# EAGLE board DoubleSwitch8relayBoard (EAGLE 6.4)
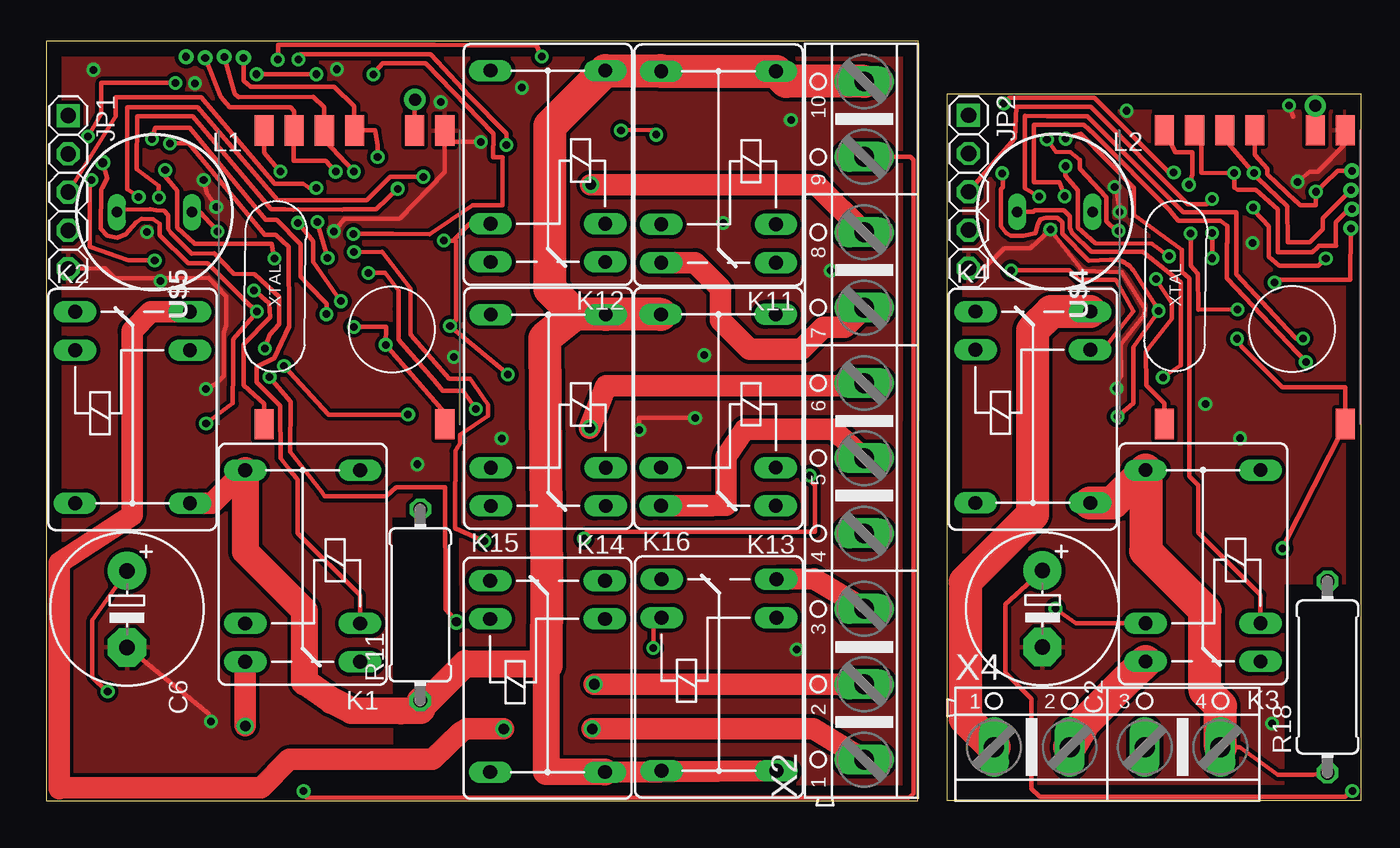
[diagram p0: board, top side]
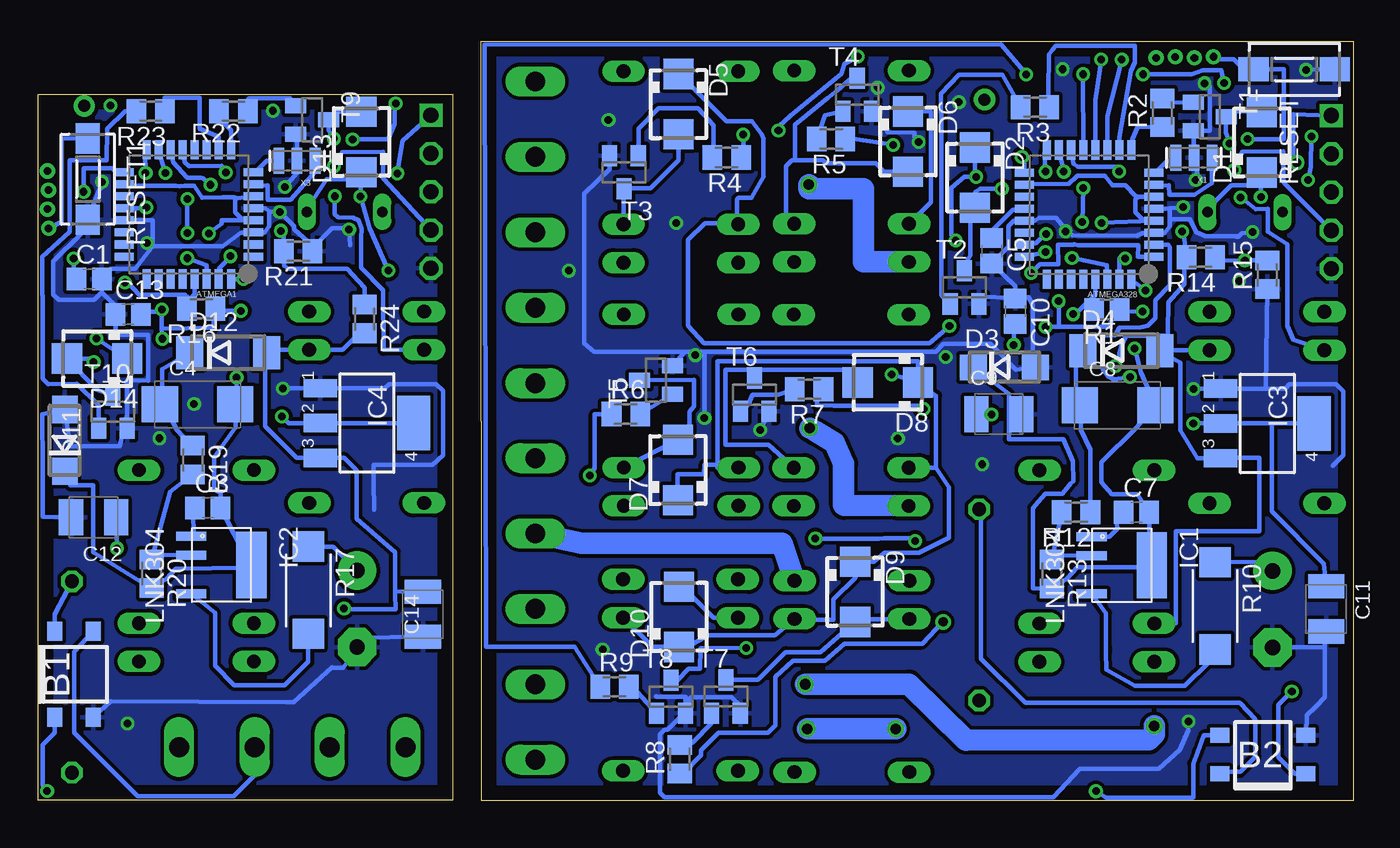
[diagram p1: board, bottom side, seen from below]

Size 87.28 x 50.4 mm. Coordinates in mm from the lower left corner, seen from the top.
Outline: 59.78,46.89 87.28,46.89 87.28,46.8 87.28,0.02 59.78,0.02 59.78,46.89
Outline: 0,0 57.85,0 57.9,50.38 0,50.4 0,0
Copper layers (1*16): Top 0.035mm / dielectric 1.5mm / Bottom 0.035mm
Design rules "default": minimum track width 10mil, minimum drill 24mil, track to track 8mil, track to pad 8mil, pad to pad 8mil, via to via 8mil, smd to smd 8mil, copper to edge 40mil, drill to drill 8mil, minimum pad ring 10mil, minimum via ring 8mil, stop-mask expansion 4mil, vias tented up to drill 0mil, thermal gap 10mil
Net classes: 1 power: width 0.381 mm, clearance 0.254 mm; 2 220V: width 0.381 mm, clearance 0.508 mm

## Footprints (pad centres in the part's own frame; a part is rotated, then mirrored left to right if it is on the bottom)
TQFP32-08 = smd 1.27 x 0.533: 1 -4.293,2.8; 2 -4.293,2; 3 -4.293,1.2; 4 -4.293,0.4; 5 -4.293,-0.4; 6 -4.293,-1.2; 7 -4.293,-2; 8 -4.293,-2.8; 17 4.293,-2.8; 18 4.293,-2; 19 4.293,-1.2; 20 4.293,-0.4; 21 4.293,0.4; 22 4.293,1.2; 23 4.293,2; 24 4.293,2.8 | smd 0.533 x 1.27: 9 -2.8,-4.293; 10 -2,-4.293; 11 -1.2,-4.293; 12 -0.4,-4.293; 13 0.4,-4.293; 14 1.2,-4.293; 15 2,-4.293; 16 2.8,-4.293; 25 2.8,4.293; 26 2,4.293; 27 1.2,4.293; 28 0.4,4.293; 29 -0.4,4.293; 30 -1.2,4.293; 31 -2,4.293; 32 -2.8,4.293
TO-269AA = smd 1 x 1.25: + -1.28,-2.855; - 1.28,-2.855; AC1 -1.28,2.855; AC2 1.28,2.855
C2012 = smd 1.3 x 1.5: 1 -0.85,0; 2 0.85,0
E5-10,5 = drill 1.016 pad 2.54: + -2.54,0 | drill 1.016 pad 2.54 octagon: - 2.54,0
SMC_C = smd 2.4 x 2.4: + -2.5,0; - 2.5,0
SMC_B = smd 1.6 x 2.4: + -1.5,0; - 1.5,0
SMA = smd 2 x 2: A 2,0; C -2,0
DO214AC = smd 1.8 x 1.7: A 2.05,0; C -2.05,0
DO214AA = smd 1.8 x 2.2: A 2.55,0; C -2.55,0
SO-8C = smd 0.6 x 2: BP -1.905,-2; D 1.905,-2; FB -0.635,-2 | smd 4.41 x 2: S 0,2
SOT223 = smd 1.219 x 2.235: 1 -2.311,-3.099; 2 0,-3.099; 3 2.311,-3.099 | smd 3.6 x 2.2: 4 0,3.099
1X05-S = drill 1.016 square: 1 -5.08,0 | drill 1.016 octagon: 2 -2.54,0; 3 0,0; 4 2.54,0; 5 5.08,0
FRS1B = drill 0.914 long: 1 0,3.81; 2 0,-3.81; O -2.54,-3.81; P 10.16,3.81; P@ 10.16,-3.81; S -2.54,3.81
BS11 = drill 0.7 long: 1 -2.5,0; 2 2.5,0
R2012 = smd 1.3 x 1.5: 1 -0.85,0; 2 0.85,0
M2012 = smd 1.3 x 1.6: 1 -0.95,0; 2 0.95,0
R2512W = smd 2 x 2.1: 1 -2.896,0; 2 2.896,0
0411/12 = drill 0.914 octagon: 1 -6.35,0; 2 6.35,0
DTSM-3 = smd 2 x 1.6: 1 -2.7,0; 2 2.7,0
SOT23 = smd 1 x 1.4: 1 -0.95,-1.1; 2 0.95,-1.1; 3 0,1.1
RFM12B-ANTENNA = drill 0.8 pad 1.422: P$1 0,0
AVRHEADER = drill 0.5: CLK 2.54,0; MISO 1.27,0.07; MOSI 0,0; VPP -1.27,0.072
RFM69W-MINPADS = smd 2 x 1.27: ANA 8,-5; DIO0 -11.5,5; GND 8,-7; MISO 8,1; MOSI 8,3; NSS 8,5; SCK 8,-1; VDD -11.5,-7
RESONATOR-SMD = smd 0.7 x 1.7: 1 -1.2,0; 2 0,0; 3 1.2,0
AK500/10 = drill 1.321 long: 1 -22.504,0; 2 -17.501,0; 3 -12.497,0; 4 -7.493,0; 5 -2.489,0; 6 2.489,0; 7 7.493,0; 8 12.497,0; 9 17.501,0; 10 22.504,0
AK500/4 = drill 1.321 long: 1 -7.518,0; 2 -2.489,0; 3 2.489,0; 4 7.518,0

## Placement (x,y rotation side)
ATMEGA1  ATMega-328  [TQFP32-08]  77.29,38.9 180 bottom
ATMEGA328  ATMega-328  [TQFP32-08]  17.52,38.88 180 bottom
B1  RECTIFIER  [TO-269AA]  84.92,8.38 0 bottom
B2  RECTIFIER  [TO-269AA]  5.99,3.05 90 bottom
C1  0.1  [C2012]  83.91,34.61 0 bottom
C2  3,3uF  [E5-10,5]  66.12,12.73 270 top
C3  100nF  [C2012]  76.03,19.42 0 bottom
C4  22uF / 16 V  [SMC_C]  76.71,26.29 0 bottom
C5  0.1  [C2012]  23.99,36.48 270 bottom
C6  3,3uF  [E5-10,5]  5.35,12.7 270 top
C7  100nF  [C2012]  14.38,19.13 0 bottom
C8  22uF / 16 V  [SMC_C]  15.64,26.24 0 bottom
C9  100uF  [SMC_B]  23.51,25.65 0 bottom
C10  100nF  [C2012]  22.43,32.48 270 bottom
C11  100uF  [SMC_B]  1.79,12.72 270 bottom
C12  100uF  [SMC_B]  83.61,18.8 180 bottom
C13  100nF  [C2012]  81.32,32.27 0 bottom
C14  100uF  [SMC_B]  61.75,12.37 270 bottom
D1  MBRA340T3  [SMA]  6.06,43.68 90 bottom
D2  MBRA340T3  [SMA]  25.1,41.34 270 bottom
D3  ES1D  [DO214AC]  23.15,28.75 0 bottom
D4  1N4007GP  [DO214AA]  15.38,29.86 0 bottom
D5  MBRA340T3  [SMA]  44.79,46.22 270 bottom
D6  MBRA340T3  [SMA]  29.55,43.73 270 bottom
D7  MBRA340T3  [SMA]  44.82,21.94 90 bottom
D8  MBRA340T3  [SMA]  30.89,27.75 180 bottom
D9  MBRA340T3  [SMA]  33.05,13.85 270 bottom
D10  MBRA340T3  [SMA]  44.74,12.19 90 bottom
D11  ES1D  [DO214AC]  85.52,23.9 90 bottom
D12  1N4007GP  [DO214AA]  74.67,29.72 0 bottom
D13  MBRA340T3  [SMA]  65.83,43.7 90 bottom
D14  MBRA340T3  [SMA]  83.37,29.34 180 bottom
IC1  LNK304  [SO-8C]  15.35,15.62 270 bottom
IC2  LNK304  [SO-8C]  75.13,15.64 270 bottom
IC3  MC33269ST-3.3T3  [SOT223]  5.69,25.03 270 bottom
IC4  MC33269ST-3.3T3  [SOT223]  65.47,25.05 270 bottom
JP1  [1X05-S]  1.44,40.38 270 top
JP2  [1X05-S]  61.22,40.4 270 top
K1  FRS1B  [FRS1B]  17.01,11.75 90 top
K2  FRS1B  [FRS1B]  5.71,29.89 270 top
K3  FRS1B  [FRS1B]  76.78,11.78 90 top
K4  FRS1B  [FRS1B]  65.49,29.92 270 top
K11  FRS1B  [FRS1B]  44.62,38.24 90 top
K12  FRS1B  [FRS1B]  33.29,38.28 90 top
K13  FRS1B  [FRS1B]  44.61,22.1 90 top
K14  FRS1B  [FRS1B]  33.32,22.09 90 top
K15  FRS1B  [FRS1B]  33.27,12.05 270 top
K16  FRS1B  [FRS1B]  44.65,12.14 270 top
L1  680uH  [BS11]  7.17,39.05 0 top
L2  680uH  [BS11]  66.94,39.07 0 top
R1  10k  [R2012]  16.34,32.59 180 bottom
R2  1 K  [M2012]  12.67,45.64 90 bottom
R3  1 K  [M2012]  21.12,46.02 180 bottom
R4  1 K  [M2012]  41.58,42.68 180 bottom
R5  1 K  [M2012]  34.65,43.91 180 bottom
R6  1 K  [M2012]  48.28,25.65 0 bottom
R7  1 K  [M2012]  36.11,27.3 180 bottom
R8  1 K  [M2012]  44.69,2.74 90 bottom
R9  1 K  [M2012]  49.03,7.55 0 bottom
R10  100  [R2512W]  9.16,12.92 270 bottom
R11  8,2  [0411/12]  24.82,12.98 90 top
R12  3.9 k  [M2012]  18.39,19.14 180 bottom
R13  2,05 k  [M2012]  19.98,15.03 270 bottom
R14  470  [M2012]  10.11,36.05 180 bottom
R15  470  [M2012]  5.69,34.89 90 bottom
R16  10k  [M2012]  76.47,32.65 180 bottom
R17  100  [R2512W]  69.35,13.96 270 bottom
R18  8,2  [0411/12]  85.05,8.2 90 top
R19  3.9 k  [M2012]  77.02,22.6 270 bottom
R20  2,05 k  [M2012]  79.76,15.06 270 bottom
R21  560  [M2012]  70.03,36.46 180 bottom
R22  1 K  [M2012]  74.33,45.75 0 bottom
R23  1 K  [M2012]  79.82,45.75 180 bottom
R24  560  [M2012]  65.61,31.96 270 bottom
RESET  [DTSM-3]  3.9,48.52 0 bottom
RESET1  [DTSM-3]  84,41.23 270 bottom
T1  BC846  [SOT23]  9.51,45.39 270 bottom
T2  BC846  [SOT23]  25.8,34.05 0 bottom
T3  BC846  [SOT23]  48.4,41.69 180 bottom
T4  BC846  [SOT23]  32.92,46.84 0 bottom
T5  BC846  [SOT23]  46.28,27.9 90 bottom
T6  BC846  [SOT23]  39.73,26.94 0 bottom
T7  BC846  [SOT23]  41.63,6.9 0 bottom
T8  BC846  [SOT23]  45.28,6.89 0 bottom
T9  BC846  [SOT23]  69.1,45.17 270 bottom
T10  BC846  [SOT23]  82.33,25.81 0 bottom
U$1  RFM12B_ANTENNA  [RFM12B-ANTENNA]  24.46,46.52 0 top
U$2  AVRHEADERDIP  [AVRHEADER]  10.54,49.29 0 top
U$3  RFM12B_ANTENNA  [RFM12B-ANTENNA]  84.24,46.1 0 top
U$4  RFM69  [RFM69W-MINPADS]  79.22,36.49 90 top
U$5  RFM69  [RFM69W-MINPADS]  19.45,36.46 90 top
U$6  AVRHEADERDIP  [AVRHEADER]  86.67,39.24 90 top
X1  16 MHz  [RESONATOR-SMD]  10.57,42.66 180 bottom
X2  [AK500/10]  54.29,25.22 90 top
X3  16 MHz  [RESONATOR-SMD]  70.1,42.46 180 bottom
X4  [AK500/4]  70.42,3.55 0 top

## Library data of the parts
ATMEGA1 ATMEGA328 U$1 U$3-U$5 = LowPowerLab
B1 B2 = rectifier
C1-C14 R1-R24 = resistor
D1-D14 = diode
IC1 IC2 = powerint
IC3 IC4 = linear
JP1 JP2 = pinhead-2
K1-K4 K11-K16 = relay; OC_FARNELL: unknown; OC_NEWARK: unknown
L1 L2 = inductor-neosid; OC_FARNELL: unknown; OC_NEWARK: unknown
RESET RESET1 = switch-tact
T1-T10 = transistor
U$2 U$6 = RemoteHome
X1 X3 = SparkFun
X2 X4 = con-ptr500; OC_FARNELL: unknown; OC_NEWARK: unknown

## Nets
5V: C14.+ D12.A D13.C D14.C IC4.3 K3.1 K4.1 L2.2 R24.2
5V1: C9.+ D1.C D2.C D4.A D5.C D6.C D7.C D8.C D9.C D10.C IC3.3 K1.1 K2.1 K11.1 K12.1 K13.1 K14.1 K15.1 K16.1 L1.2 R14.2
A0: ATMEGA328.23 R9.1
A1: ATMEGA328.24 R6.1
A2: ATMEGA328.25
A3: ATMEGA328.26
A4: ATMEGA1.22
A4_SDA: ATMEGA328.27
A4_SDA1: ATMEGA1.27
A5: ATMEGA1.19
A5_SCL: ATMEGA328.28
A5_SCL1: ATMEGA1.28
A6: ATMEGA328.19
A7: ATMEGA328.22
A8: ATMEGA1.26
A9: ATMEGA1.25
A10: ATMEGA1.24
A11: ATMEGA1.23
AREF: ATMEGA328.20 C5.1
AREF1: ATMEGA1.20 C1.1
D0_RX: ATMEGA328.30 JP1.3
D0_RX1: ATMEGA1.30 JP2.3
D1: ATMEGA1.13 R21.2 R24.1
D1_TX: ATMEGA328.31 JP1.4
D1_TX1: ATMEGA1.31 JP2.4
D2: ATMEGA328.32 U$5.DIO0
D3: ATMEGA328.1 R7.1
D4: ATMEGA328.2 R8.1
D5: ATMEGA328.9 R2.1
D6: ATMEGA328.10 R3.1
D7: ATMEGA328.11 R4.1
D8: ATMEGA328.12 R5.1
D9: ATMEGA328.13 R14.1 R15.2
D10: ATMEGA1.12
D10_SS: ATMEGA328.14 U$5.NSS
D10_SS1: ATMEGA1.14 U$4.NSS
D11: ATMEGA1.11
D11_MOSI: ATMEGA328.15 U$2.MOSI U$5.MOSI
D11_MOSI1: ATMEGA1.15 U$4.MOSI U$6.MOSI
D12: ATMEGA1.10 R23.1
D12_MISO: ATMEGA328.16 U$2.MISO U$5.MISO
D12_MISO1: ATMEGA1.16 U$4.MISO U$6.MISO
D13: ATMEGA1.9 R22.1
D13_SCK: ATMEGA328.17 U$2.CLK U$5.SCK
D13_SCK1: ATMEGA1.17 U$4.SCK U$6.CLK
D14: ATMEGA1.2
D15: ATMEGA1.1
D16: ATMEGA1.32 U$4.DIO0
GND [power]: ATMEGA328.3 ATMEGA328.5 ATMEGA328.21 B2.- C5.2 C6.- C9.- C10.1 C11.- D3.A IC3.1 JP1.5 R15.1 RESET.2 T1.2 T2.2 T3.2 T4.2 T5.2 T6.2 T7.2 T8.2 U$5.GND X1.2
GND1 [power]: ATMEGA1.3 ATMEGA1.5 ATMEGA1.21 B1.- C1.2 C2.- C12.- C13.1 C14.- D11.A IC4.1 JP2.5 R21.1 RESET1.2 T9.2 T10.2 U$4.GND X3.2
N678: IC2.FB R19.2 R20.1
N$1: ATMEGA328.7 X1.1
N$2: R2.2 T1.1
N$3: U$1.P$1 U$5.ANA
N$4: D2.A K2.2 T2.3
N$5: D1.A K1.2 T1.3
N$6: R3.2 T2.1
N$7 [220V]: K1.S X2.2
N$8 [220V]: K12.P
N$9 [220V]: B2.AC2 X2.9
N$10: C7.2 C8.- D3.C IC1.S L1.1 R13.2
N$11 [220V]: K1.P@
N$12: ATMEGA1.7 X3.1
N$13 [220V]: IC1.D R10.2
N$14 [220V]: B2.+ C6.+ R10.1
N$15 [220V]: B2.AC1 R11.2
N$16 [220V]: K2.P@
N$17 [220V]: K1.O
N$18: C7.1 IC1.BP
N$19 [220V]: K2.O
N$20: C8.+ D4.C R12.1
N$21: ATMEGA328.8 X1.3
N$22: D5.A K11.2 T3.3
N$23: ATMEGA1.8 X3.3
N$24: R4.2 T3.1
N$25: D6.A K12.2 T4.3
N$26: R5.2 T4.1
N$27: D7.A K13.2 T5.3
N$28: R6.2 T5.1
N$29: D8.A K14.2 T6.3
N$30: R7.2 T6.1
N$31: D9.A K15.2 T7.3
N$32: R8.2 T7.1
N$33: D10.A K16.2 T8.3
N$34: R9.2 T8.1
N$35 [220V]: K14.P
N$36 [220V]: K12.S X2.8
N$37 [220V]: K11.S X2.7
N$38 [220V]: K13.P@
N$39: U$3.P$1 U$4.ANA
N$40 [220V]: K15.P@
N$41 [220V]: K1.P K2.P K11.P K11.P@ K12.P@ K13.P K14.P@ K15.P K16.P K16.P@ R11.1 X2.10
N$42 [220V]: K11.O
N$43 [220V]: K12.O
N$44 [220V]: K13.O
N$45 [220V]: K14.O
N$46 [220V]: K15.O
N$47 [220V]: K16.S X2.3
N$48 [220V]: K2.S X2.1
N$49 [220V]: K3.P K4.P R18.1 X4.4
N$50 [220V]: K13.S X2.5
N$51 [220V]: K14.S X2.6
N$52 [220V]: K15.S X2.4
N$53 [220V]: K16.O
N$54 [220V]: B1.AC2 X4.3
N$55 [220V]: K3.S X4.2
N$56 [220V]: IC2.D R17.2
N$57 [220V]: B1.+ C2.+ R17.1
N$58 [220V]: B1.AC1 R18.2
N$59: C3.1 IC2.BP
N$60: C4.+ D12.C R19.1
N$61: D13.A K3.2 T9.3
N$62: R22.2 T9.1
N$63: C3.2 C4.- D11.C IC2.S L2.1 R20.2
N$64: D14.A K4.2 T10.3
N$65: R23.2 T10.1
N$66 [220V]: K4.S X4.1
N$67 [220V]: K3.P@
N$68 [220V]: K4.P@
N$69 [220V]: K3.O
N$70 [220V]: K4.O
RST: ATMEGA328.29 R1.2 RESET.1 U$2.VPP
RST1: ATMEGA1.29 R16.2 RESET1.1 U$6.VPP
VCC: ATMEGA328.4 ATMEGA328.6 ATMEGA328.18 C10.2 C11.+ IC3.2 IC3.4 JP1.1 R1.1 U$5.VDD
VCC1: ATMEGA1.4 ATMEGA1.6 ATMEGA1.18 C12.+ C13.2 IC4.2 IC4.4 JP2.1 R16.1 U$4.VDD
XXX: IC1.FB R12.2 R13.1

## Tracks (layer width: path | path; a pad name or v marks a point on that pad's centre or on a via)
5V  (via drill 0.5)
  Top 0.305: K3.1 68.35,11.78 v66.98,12.74 | v65.9,40.09 64.95,40.63 64.95,45.44 66.42,45.42 69.12,45.42 75.47,39.03 78.98,39.03 78.99,34.94 82.36,31.27 82.97,30.66 v83.41,30.66 | v64.05,35.19 67.92,35.19 68.53,34.57 70.95,34.57 71.04,34.48 72.15,32.48 70.14,29.88 K4.1
  Bottom 0.305: 63.6,13.88 63.6,13.71 63.55,12.7 66.91,12.7 66.96,12.72 v66.98,12.74 | 63.6,13.88 63.6,16.49 66.14,18.69 66.14,21.93 66.97,22.75 68.56,22.75 IC4.3 70.12,22.74 72.21,24.83 72.21,29.64 D12.A 71.93,29.91 K4.1 67.08,29.91 65.98,31.01 R24.2 | 65.9,40.89 v65.9,40.09 65.3,37.98 v64.04,35.19 v64.05,35.19 | 65.9,40.89 D13.C | 65.9,40.89 65.91,41.24 68.13,41.24 69.44,39.27 L2.2 | D14.C v83.41,30.66 | C14.+ 63.6,13.88
5V1  (via drill 0.5)
  Top 0.305: v11.36,37.77 11.24,37.9 10.19,39.05 L1.2 | v24.01,25.61 22.24,25.61 18.75,25.61 v15.78,28.84 | v25.03,41.4 24.08,41.4 23.14,41.41 22.82,41.41 21.27,39.84 15.35,39.84 10.06,46.02 6.65,46.02 5.36,46 5.37,40.58 v6.12,40.06 | K12.1 28.1,38.28 26.98,37.17 v26.39,37.17 27.17,37.17 27.2,37.14 27.2,31.88 27.18,31.86 26.83,31.53 v26.8,31.49 v30.64,28.28
  Bottom 0.305: D4.A 11.47,29.04 11.47,24.56 10.34,22.72 IC3.3 8.79,22.74 6.23,22.74 6.23,17.89 11.75,17.89 11.75,11.75 K1.1 | 12.9,29.89 D4.A | v11.36,37.77 11.19,37.24 R14.2 11.21,36.2 11.2,34.28 12.28,33.08 12.3,31.16 12.37,30.24 | 12.37,30.24 12.39,29.88 D4.A | C9.+ v24.01,25.61 | v15.78,28.84 15.52,28.71 15.5,29.04 15.52,29.7 15.35,30.28 15.06,30.85 12.37,30.84 12.37,30.24 | D4.A | v6.12,40.06 6.12,40.87 | L1.2 9.67,39.25 8.1,40.82 6.17,40.82 6.12,40.87 | v26.39,37.17 26.65,37.5 26.65,40.66 25.79,41.4 v25.03,41.4 25.1,41.8 D2.C | D6.C 28.02,45.72 28.02,43.31 28.02,39.7 K12.1 | D5.C 44.68,48.17 41.6,45.09 39.91,45.09 39.24,44.2 39.13,43.92 39.13,42.47 39.13,41.4 39.94,40 40.79,40 40.88,39.91 40.88,38.31 K11.1 40.89,38.32 43.03,38.32 44.14,37.2 44.14,31.51 43.1,30.35 33.1,30.36 33.1,30.35 28.12,30.35 v26.8,31.49 | D1.C 6.06,40.93 6.12,40.87 | K2.1 12.79,29.89 D4.A | 27.68,22.09 27.68,26.87 28.89,27.72 D8.C | K13.1 42.2,22.1 42.2,22.29 | 42.2,22.29 42.2,29.17 28.89,29.17 D8.C | D7.C 44.85,21.65 43.1,21.65 43.05,22.29 42.2,22.29 | K16.1 46.52,10.19 D10.C 44.17,10.19 42.8,10.98 38.37,10.98 K15.1 37.02,12 34.95,12 34.51,11.99 34.51,13.37 33.05,14.78 33.05,14.96 D9.C 31.8,15.85 31.12,16.43 28.82,16.43 26.83,17.44 26.83,20.78 27.68,22.09 | K14.1 27.68,22.09 | v30.64,28.28 D8.C
A0  (via drill 0.5)
  Top 0.305: v20.39,37.6 23.02,37.6 25.45,37.59 28.3,39.52 30.27,39.52 30.27,42.69 29.65,42.69 29.67,44.26 25.16,48.92 22.32,48.92 v21.7,48.19
  Bottom 0.305: ATMEGA328.23 21.07,37 v20.39,37.6 | v21.7,48.19 23.37,50.2 57.67,50.15 57.57,10.22 51.68,10.22 R9.1
A1  (via drill 0.5)
  Top 0.305: v20.42,36.4 22.3,36.41 24.18,33.96 24.17,30.92 26.73,27.98 28.11,27.98 29.31,26.28 29.32,25.52 27.45,24.28 27.45,23.72 27.3,23.45 27.15,23.21 27.14,19.15 27.14,18.08 v29.06,17.22 | v35.69,17.39 35.85,17.83 51,17.83 51,20.91 50.67,21.25 v50.67,21.58
  Bottom 0.305: ATMEGA328.24 v20.42,36.4 | v29.06,17.22 29.4,17.4 31.15,17.4 31.47,17.38 35.12,17.38 v35.69,17.39 | R6.1 50.34,25.64 50.34,22.09 50.6,21.54 v50.67,21.58
AREF
  Bottom 0.305: C5.1 24,37.33 24.01,37.34 24.01,37.78 23.41,38.38 | 23.41,38.38 | 23.41,38.38 22.58,39.21 21.88,39.21 ATMEGA328.20
AREF1  (via drill 0.5)
  Top 0.305: v80.12,39.36 80.17,39.19 81.16,38.11 81.16,36.1 81.83,35.51 84.44,35.51 v84.93,35.97
  Bottom 0.305: ATMEGA1.20 80.42,39.3 v80.12,39.36 | v84.93,35.97 84.95,34.81 C1.1
D0_RX  (via drill 0.5)
  Top 0.305: v17.91,40.65 17.43,40.65 17.04,40.94 15.16,40.92 10.29,46.66 4.61,46.68 4.59,45.43 JP1.3 | v17.98,38.39 v18.66,36.02
  Bottom 0.305: v17.91,40.65 v17.98,38.39 | v18.66,36.02 16.34,35.52 ATMEGA328.30
D0_RX1  (via drill 0.5)
  Top 0.305: v77.38,37.66 v77.39,35.99 | JP2.3 64.29,43.96 64.39,46.03 69.35,46.04 75.76,39.56 75.78,39.58 77.05,39.58 77.38,39.91 v77.38,39.93
  Bottom 0.305: v77.38,39.93 v77.38,37.66 | v77.39,35.99 76.12,35.54 ATMEGA1.30
D1  (via drill 0.5)
  Top 0.305: v71.19,37.81 71.02,37.83 70.36,38.45 70.38,40.04 68.6,41.93 68.6,42.51 67.97,43.03 67.02,43.05 v66.42,43.88 | v63.56,46.26 | v63.56,46.26 63.93,46.63 69.58,46.63 74.52,41.71 v74.84,41.69
  Bottom 0.305: R24.1 65.61,34.04 66.77,35.3 70.68,35.3 70.96,35.48 70.96,36.22 R21.2 70.98,38 v71.19,37.81 | v66.42,43.88 64.07,43.88 63.61,44.93 63.61,46.21 v63.56,46.26 | ATMEGA1.13 77.55,42.37 77.28,42.1 75.11,42.12 v74.84,41.69
D1_TX  (via drill 0.5)
  Top 0.305: v7.88,41.83 7.88,41.43 8.69,40.47 8.69,38 9.85,36.95 14.94,36.95 v15.12,35.98
  Bottom 0.305: v7.88,41.83 7.34,43.07 4.64,43.09 4.62,41.06 4.57,40.98 JP1.4 | v15.12,35.98 15.5,36 15.51,35.56 15.51,34.6 ATMEGA328.31
D1_TX1  (via drill 0.5)
  Top 0.305: v67.66,42.1 67.66,41.45 68.46,40.49 68.46,38.02 69.63,36.97 73.4,36.96 v74.53,36.13
  Bottom 0.305: v67.66,42.1 67.12,43.04 64.39,43.06 64.39,41.3 JP2.4 | v74.53,36.13 75.02,35.58 75.28,35.32 ATMEGA1.31
D2  (via drill 0.5)
  Top 0.305: U$5.DIO0 14.45,26.34 13.1,27.56 13.1,30.29 14.84,32.07 14.8,33 v13.78,33.86
  Bottom 0.305: v13.78,33.86 14.71,34.58 ATMEGA328.32
D3  (via drill 0.5)
  Top 0.305: v21.36,35.02 22.48,35.02 23.39,33.83 23.37,32.61 23.38,30.57 24.27,29.57 25.75,27.89 26.3,27.2 27.66,27.19 v28.52,25.98
  Bottom 0.305: ATMEGA328.1 14.28,36.08 14.27,36.87 18.27,36.87 18.51,36.92 18.57,36.88 19.58,36.89 19.57,35.59 20.02,35.59 20.8,35.59 v21.36,35.02 | v28.52,25.98 28.71,26.2 30.77,26.19 34.42,26.19 34.49,26.19 35.57,26.22 35.57,27.26 R7.1
D4  (via drill 0.5, 0.6)
  Top 0.305: v14.81,28.1 16.2,26.47 16.19,23.15 18.26,20.49 18.45,20.19 22.54,20.19 23.2,20.79 26.48,20.79 26.49,12.7 v27.21,11.85
  Bottom 0.305: R8.1 44.49,1.79 43.29,3 43.29,3.35 42.14,4.5 38.83,4.5 38.35,4.99 38.35,8.2 37.19,9.29 35.07,9.29 33.77,10.41 28.59,10.41 v27.21,11.85 | ATMEGA328.2 12.27,36.88 12.16,36.72 12.16,34.21 13.11,33.2 13.11,32 13.62,31.49 14.09,31.4 15.53,31.37 15.77,30.87 16.6,30.86 16.62,28.58 16.29,28.15 15.89,27.96 v14.81,28.1
D5
  Bottom 0.305: R2.1 13.88,44.7 14.29,44.7 14.66,43.89 ATMEGA328.9
D6
  Bottom 0.305: ATMEGA328.10 15.52,44.02 14.75,48.39 14.49,49.01 14.49,50.09 17.53,50.09 19.72,50.09 19.97,49.83 20.21,49.51 20.21,47.09 R3.1
D7  (via drill 0.5)
  Top 0.305: v15.35,49.17 15.38,49.35 15.38,50.14 20.41,50.14 21.87,50.15 25.76,50.15 27.76,50.13 32.53,50.13 v32.88,49.37 | v38.15,44.48 40.46,44.53 v40.48,44.19
  Bottom 0.305: ATMEGA328.11 16.32,45.4 v15.35,49.17 | v32.88,49.37 33.77,48.88 33.97,48.22 37.36,45.44 38.13,44.77 v38.15,44.48 | v40.48,44.19 40.48,43.2 R4.1
D8  (via drill 0.5)
  Top 0.305: v16.72,49.18 16.75,49.33 16.8,49.52 25.52,49.52 28.11,46.76 30.55,44.26 v30.52,43.51
  Bottom 0.305: ATMEGA328.12 17.12,46.47 v16.72,49.18 | v30.52,43.51 33.18,43.93 R5.1
D9  (via drill 0.5)
  Top 0.305: v7.18,35.84 5.41,35.84 2.89,36.74 2.89,40.62 v2.98,41.19 | v2.77,44.08 3.64,45.58 3.64,47.63 v8.57,47.63 | v17.92,48.2 v13.95,48.2
  Bottom 0.305: 8.8,35.84 R14.1 8.88,35.83 v7.18,35.84 R15.2 | v2.98,41.19 2.8,42.07 v2.77,44.08 | ATMEGA328.13 v17.92,48.2 | v13.95,48.2 10.71,48.2 9.98,48.47 8.75,48.47 v8.57,47.63
D10_SS  (via drill 0.5)
  Top 0.305: U$5.NSS 14.45,42.98 v15.53,41.74
  Bottom 0.305: v15.53,41.74 15.71,42.07 17.07,42.05 18.25,42.05 18.55,42.27 18.7,43.16 ATMEGA328.14
D10_SS1  (via drill 0.5)
  Top 0.305: U$4.NSS 74.94,43.02 76.07,43.02 76.09,41.54 v75.84,40.87
  Bottom 0.305: v75.84,40.87 76.33,41.29 76.47,41.34 77.41,41.34 78.32,42.36 78.48,43.18 ATMEGA1.14
D11_MOSI  (via drill 0.5)
  Top 0.305: v19.2,41.73 18.55,42.46 16.42,42.45 U$5.MOSI 16.46,44.48 16.46,45.73 16.23,46 12.17,46.01 11.57,46.71 U$2.MOSI
  Bottom 0.305: v19.2,41.73 19.54,43.15 ATMEGA328.15
D11_MOSI1  (via drill 0.5)
  Top 0.305: U$4.MOSI 76.67,43.67 76.67,41.67 v78.83,41.64 78.85,41.63 78.85,40.67 79.09,40.53 80.3,40.53 81.74,39.23 81.74,36.4 84.02,36.38 84.38,36.72 84.47,36.81 85.62,36.81 85.59,36.84 85.59,38.37 86.46,39.24 U$6.MOSI
  Bottom 0.305: v78.83,41.64 79.32,43.17 ATMEGA1.15
D12
  Bottom 0.305: ATMEGA1.10 75.29,44.05 76.56,44.58 76.56,46.64 78.88,46.64 78.89,45.81 R23.1
D12_MISO  (via drill 0.5)
  Top 0.305: v20.42,41.73 18.45,43.85 U$5.MISO 18.43,44.48 18.43,46 17.7,46.71 12.74,46.69 12.49,46.92 U$2.MISO
  Bottom 0.305: v20.42,41.73 20.49,43 ATMEGA328.16
D12_MISO1  (via drill 0.5)
  Top 0.305: U$4.MISO 78.22,43.88 v80.15,41.64 v80.16,41.65 80.42,41.29 82.39,39.44 82.39,37.05 83.85,37.05 84.73,37.93 84.73,38.64 U$6.MISO
  Bottom 0.305: v80.15,41.64 80.19,43.02 ATMEGA1.16
D13
  Bottom 0.305: 74.54,43.25 ATMEGA1.9 74.49,44.49 75.28,45.28 R22.1
D13_SCK  (via drill 0.5)
  Top 0.305: v21.98,42.72 21.98,43.51 21.82,44.47 U$5.SCK 20.44,46.09 19.08,47.38 13.57,47.38 13.08,47.76 U$2.CLK
  Bottom 0.305: ATMEGA328.17 21.81,42.84 v21.98,42.72
D13_SCK1  (via drill 0.5)
  Top 0.305: U$4.SCK 80.23,42.85 81.05,41.94 81.05,41.56 82.94,39.76 83,39.73 83.25,39.51 84.26,39.51 v84.27,40.4 85.61,41.67 85.73,41.79 U$6.CLK
  Bottom 0.305: ATMEGA1.17 82.11,41.7 82.38,41.97 84.25,41.95 v84.27,40.4
D16  (via drill 0.5)
  Top 0.305: U$4.DIO0 74.22,26.36 73.02,27.57 72.99,29.78 74.69,31.97 74.69,33.02 v73.66,34.6
  Bottom 0.305: v73.66,34.6 ATMEGA1.32
GND  (via drill 0.5)
  Top 0.305: U$5.GND 26.45,43.89 | 26.45,43.89 26.45,41.71 23.44,38.61 19.8,38.61 v19.08,37.78 | v10.59,27.32 11.28,27.67 11.75,28.14 11.75,31.06 11.93,31.56 11.93,33.45 10.78,34.7 8.7,34.67 8.69,34.67 4.52,34.67 3.86,35.32 3.75,35.32 JP1.5 | v10.44,41.18 10.63,40.32 v11.27,39.4 | v28.83,43.72 26.52,43.71 26.45,43.89 | v39.35,24.59 39.35,25.4 v43.06,25.4 | v10.92,5.25 10.76,5.75 C6.-
  Bottom 0.305: 5.74,27.34 IC3.1 10.39,27.34 v10.59,27.32 | 5.74,27.34 4.5,27.34 4.22,27.62 1.1,27.62 0.65,27.16 0.65,22.9 1.33,22.22 | 10.58,44.26 X1.2 10.33,41.65 v10.44,41.18 | C10.1 22.43,34.15 C5.2 22.87,36.75 22.87,38.13 22.52,38.48 ATMEGA328.21 21.16,38.48 20.84,38.68 19.74,38.66 18.9,37.72 18.63,37.51 14.34,37.49 13.99,37.66 13.24,37.66 ATMEGA328.3 13.21,37.66 12.53,37.66 12.15,38.11 12.18,38.59 | C10.1 24.35,33.45 | C10.1 22.43,33.44 22.39,33.41 21.53,33.41 21.26,32.85 21.26,29 D3.A 22.37,28.6 24.07,30.3 27.2,30.33 27.68,29.79 27.77,29.77 43.05,29.77 | ATMEGA328.5 12.45,39.28 12.17,39.3 | 12.17,39.3 12.15,38.87 12.18,38.59 | 7.62,37.44 9.77,37.45 10.39,37.71 10.85,38.59 12.18,38.59 | v11.27,39.4 11.68,39.35 12.17,39.3 | T4.2 32.09,45.6 31.06,44.89 30.89,44.36 29.1,44.32 29.1,43.86 v28.83,43.72 | T3.2 49.35,41.9 51.07,40.26 51.07,30.36 50.4,29.77 44.35,29.77 | 44.35,29.77 43.05,29.77 | T6.2 v39.35,24.59 | v43.06,25.4 43.05,29.77 | T5.2 44.35,29.77 | B2.- 3.09,4.94 3.07,5.17 3.07,5.68 2.48,6.23 1.86,6.84 1.86,10.22 C11.- 1.89,10.17 C6.- | T7.2 40.68,6.28 41.26,6.86 43.96,6.86 | 43.96,6.86 44.33,6.49 | 44.33,6.49 T8.2 | 43.96,6.86 43.97,6.86 43.97,6.27 45.52,4.71 45.7,4.71 46.02,4.39 46.02,0.53 45.7,0.21 19.89,0.21 18.14,2.11 12.9,2.11 11.49,3.38 10.92,4.68 v10.92,5.25 | RESET.2 1.78,48.52 v3.12,48.5 | v9.86,47.6 9.5,47.39 9.5,44.45 T1.2 | R15.1 5.79,27.39 5.74,27.34 | v6.67,37.74 7.39,37.65 7.62,37.43 | 7.62,37.43 7.62,37.41 | 7.62,37.43 7.62,37.44 7.6,37.46 | 7.6,37.46 | 7.6,37.46 7.63,37.43 7.74,37.43 | 44.33,6.49 44.33,6.89 46.21,6.89 46.26,6.92
  other vias: 49.43,45.18 44.93,38.34 52.06,35.16 49.82,10.03 19.28,48.53 26.17,46.35 24.62,22.32 7.56,34.49 43.68,29.56 31.56,47.31 27.05,29.43 30.22,24.03
  pour Top: 27,50.17 0.15,50.23 0.2,46.62 0.2,0.22 22.88,0.2 22.83,18.91 27.44,18.97 27.51,18.97 27.6,0.19 57.68,0.19 57.73,50.13 32.49,50.19
  pour Bottom: 25.19,50.18 0.2,50.21 0.2,0.2 57.67,0.2 57.76,42.84 57.76,50.19
GND1  (via drill 0.5)
  Top 0.305: v71.05,27.34 71.05,27.69 71.36,28.19 71.34,30.3 72.89,32.26 72.9,32.62 71.4,35.06 68.78,35.15 v66.65,37.89 65.3,36.66 63.58,36.66 62.24,35.32 JP2.5 | v70.91,40.71 71.01,40.56 v71.26,39.06 | U$4.GND 86.22,43.57 84.38,41.73 83.85,41.73 v83.05,41.06 | v82.49,46.14 82.77,45.38
  Bottom 0.305: B1.- 82.47,6.58 70.82,6.52 70.32,6.51 67.77,8.85 67.76,8.82 67.04,8.81 66.12,10.04 C2.- 66.12,10.8 C14.- | 65,19.31 65.03,21.21 65.03,22.27 61.11,22.27 60.42,22.93 60.42,27.19 60.88,27.64 64,27.64 64.28,27.36 IC4.1 71.03,27.36 v71.05,27.34 | T9.2 70.1,44.28 X3.2 70.1,41.67 v70.91,40.71 | ATMEGA1.21 79.69,38.51 79.68,36.8 | 79.68,36.8 75.04,36.78 73.88,37.64 73.77,37.69 73.02,37.69 ATMEGA1.3 72.98,37.69 72.3,37.69 71.96,38.13 71.95,38.61 71.96,39.07 71.9,39.07 | ATMEGA1.5 72.23,39.3 71.9,39.07 | 66.58,36.86 v66.65,37.89 66.64,38 67.78,38 69.08,36.7 R21.1 69.08,36.83 70.31,37.91 70.31,38.13 v71.26,39.06 71.45,39.08 71.9,39.07 | 79.68,36.8 80.85,35.3 82.48,35.3 82.86,34.84 C1.2 83.06,33.72 | 83.06,33.72 82.14,32.8 C13.1 82.14,32.55 82.14,30.92 79.99,30.91 79.99,27.86 81.39,27.89 81.39,27.91 T10.2 81.38,25.63 81.86,23.52 85.18,23.52 D11.A 87.02,25.64 87.02,25.36 87,22.45 87,18.84 C12.- | 83.06,33.72 83.56,33.22 85.94,33.22 86.28,33.57 86.28,35.78 84.51,37.55 RESET1.2 v83.05,41.06 83.12,40.64 83.15,40.61
  other vias: 81.37,5.11 71.71,45.78 76.94,26.32 79.24,24.05 80.08,37
  pour Top: 59.94,46.73 87.12,46.73 87.12,14.48 82.06,14.48 82.06,0.17 59.93,0.17 59.93,46.65
  pour Bottom: 60,46.72 87.13,46.68 87.13,0.18 59.95,0.18 59.93,46.68
N678
  Bottom 0.305: IC2.FB 77.96,16.27 79.22,16.31 79.47,16.31 R20.1 78.52,20.49 R19.2
N$1
  Bottom 0.305: ATMEGA328.7 13.22,40.84 13.18,40.79 12.23,40.82 12.18,40.19 10.54,40.21 9.38,40.96 9.38,42.19 X1.1
N$2
  Bottom 0.305: R2.2 12.3,46.31 T1.1
N$3
  Top 0.305: U$5.ANA 24.45,46.06 U$1.P$1
N$4  (via drill 0.5)
  Top 0.305: v7.47,40.03 7.45,40.81 6.65,41.41 6,41.89 6.02,45.42 8.43,45.41 8.88,45.41 9.71,45.41 14.91,39.23 15.71,39.23 15.86,39.23 16.37,39.22 16.7,39.23 19.62,39.22 19.73,39.23 21.89,39.23 v23.32,40.6
  Bottom 0.305: T2.3 25.8,35.51 25.41,36.2 25.41,38.67 25.75,39.33 D2.A 25.09,39.35 25.09,40.41 24.75,40.6 v23.32,40.6 | K2.2 3.95,30.59 4.35,31.51 4.36,36.94 5.66,37.77 5.66,38 5.66,39.28 6.45,39.25 v7.47,40.03
N$5  (via drill 0.5)
  Top 0.305: K1.2 20.82,13.63 16.69,17.76 16.69,21.28 16.12,22 15.54,22.73 15.51,26.21 13.95,27.75 13.96,28.78 15.1,29.35 16.1,31.48 16.08,36.77 15.21,37.55 14.47,37.54 9.45,43.62 8.68,43.63 v8.2,43.61
  Bottom 0.305: v8.2,43.61 8.45,44.35 T1.3 7.73,45.73 D1.A
N$6
  Bottom 0.305: R3.2 23.29,48.16 26.16,48.18 27.34,46.91 27.34,44.28 27.34,33.54 T2.1
N$7  (via drill 0.7)
  Top 1.422: X2.2 v36.36,7.72 | v13.19,4.96 K1.S
  Bottom 1.422: v36.36,7.72 29.48,7.72 25.71,4 13.56,4.02 13.19,4.39 v13.19,4.96
N$9  (via drill 0.5)
  Top 0.305: X2.9 57.37,42.72 57.57,42.52 57.57,0.45 57.23,0.19 52.41,0.19 17.28,0.2 17.07,0.41 v17.07,0.62
  Bottom 0.305: B2.AC2 9.9,4.33 10.31,3.23 10.62,2.44 10.62,0.21 10.65,0.18 16.36,0.18 v17.07,0.62
N$10  (via drill 0.5)
  Top 0.305: L1.1 4.9,39.28 5.12,39.21 6.86,39.23 6.91,39.25 7.29,39.17 7.82,39.13 8.07,38.86 8.08,37.96 8.26,37.69 9.63,36.3 11.12,36.31 12.43,34.96 13.81,34.91 15.46,33.43 15.46,31.62 14.8,30.92 v14.5,29.99
  Bottom 0.305: v14.5,29.99 14.08,28.41 C8.- 14.39,24.74 16.69,22.44 16.69,21.11 16,20.32 14.33,20.32 C7.2 13.56,15.83 IC1.S 13.48,15.49 18.3,15.49 19.03,14.68 R13.2 20,14.07 21.24,14.1 21.24,19.41 20.91,19.82 20.43,20.36 19.3,20.36 18.74,21.05 18.57,21.19 18.6,22.51 19.22,23.98 19.53,23.99 21.05,23.99 22.86,23.99 22.86,25.64 22.86,27.01 D3.C
N$12
  Bottom 0.305: ATMEGA1.7 73,40.86 72.95,40.81 72.05,40.85 72.06,39.87 70.53,39.88 68.9,41.73 X3.1
N$13
  Bottom 0.305: R10.2 9.58,9.19 11.15,7.64 14.49,7.64 16.39,8.67 16.39,9.84 16.4,10.16 16.39,12.45 IC1.D
N$14  (via drill 0.5)
  Top 0.305: v4.07,7.24 4,7.24 3.05,8.2 3.05,11.95 C6.+
  Bottom 0.305: R10.1 6.3,15.84 C6.+ | B2.+ 3.87,1.77 4.96,2.86 4.96,6.35 v4.07,7.24
N$15
  Bottom 0.305: B2.AC1 8.85,1.83 8.77,1.91 7.5,1.91 6.48,2.92 6.48,5.4 7.52,6.49 21.75,6.49 24.72,9.4 24.72,19.23 R11.2
N$18
  Bottom 0.305: C7.1 15.74,19.14 15.66,18.02 16.16,17.52 IC1.BP
N$20
  Bottom 0.305: R12.1 17.44,22.77 17.43,23.29 18.08,24.6 C8.+ 18.35,26.09 18.41,26.59 18.41,29.11 D4.C
N$21
  Bottom 0.305: ATMEGA328.8 13.11,41.68 12.35,42.44 11.53,42.44 X1.3
N$22
  Bottom 0.305: K11.2 48.43,40.56 T3.3 48.36,40.63 46.65,40.63 44.79,42.49 D5.A
N$23
  Bottom 0.305: ATMEGA1.8 72.89,41.7 72.13,42.46 X3.3 | X3.3
N$24
  Bottom 0.305: T3.1 47.45,44.6 46.11,45.94 43.47,45.94 42.45,44.82 42.45,43.18 R4.2
N$25
  Bottom 0.305: D6.A 31.13,41.73 31.67,42.28 34.98,42.28 35.2,42.5 36.77,42.5 | 36.77,42.5 37.26,42.5 37.66,42.1 37.66,38.85 K12.2 | T4.3 33.4,47.86 34.31,47.08 34.88,46.64 37.03,44.85 37.03,42.5 36.77,42.5
N$26
  Bottom 0.305: R5.2 35.06,45.48 T4.1
N$27
  Bottom 0.305: T5.3 43.74,27.92 43.74,26.16 44.05,25.81 44.05,23.69 D7.A K13.2
N$28
  Bottom 0.305: T5.1 R6.2
N$29
  Bottom 0.305: D8.A 33.38,27.33 33.74,27.33 33.74,28.6 40.16,28.6 | 40.16,28.6 41.65,28.6 41.65,23.61 38.8,23.61 K14.2 | T6.3 40.08,28.52 40.16,28.6
N$30
  Bottom 0.305: T6.1 41.03,25.39 40.14,26.3 | 40.14,26.3 | 40.14,26.3 39.88,26.95 38.18,26.95 R7.2
N$31
  Bottom 0.305: K15.2 31.42,12.04 33.07,12.03 D9.A 35.34,9.84 37.66,9.86 39.52,8.02 T7.3
N$32
  Bottom 0.305: T7.1 42.58,5.12 43.86,3.84 44.55,3.84 R8.2
N$33  (via drill 0.5)
  Top 0.305: v40.3,10.13 40.3,11.59 K16.2
  Bottom 0.305: K16.2 42.46,12.14 44.08,13.76 44.31,13.76 D10.A | v40.3,10.13 43.31,10.11 43.34,8.76 44.11,8.76 44.85,7.99 T8.3
N$34
  Bottom 0.305: R9.2 47.84,7.55 T8.1
N$36  (via drill 0.7)
  Top 1.422: v36.13,40.87 51.13,40.87 X2.8
  Bottom 1.422: K12.S 32.51,35.74 32.51,40.59 36.13,40.59 v36.13,40.87
N$37
  Top 1.422: K11.S 43.06,35.7 44.74,34.01 44.74,31.88 46.69,29.93 50.11,29.93 51.6,31.42 53,31.42 X2.7
N$39
  Top 0.305: U$4.ANA 84.22,46.08 U$3.P$1
N$41
  Top 0.305: K16.P@ K15.P
  Top 1.422: K2.P 11.02,19.73 K1.P | K16.P K15.P | 24.86,5.97 24.86,6.14 | 33.09,9.09 33.18,9
  Top 1.778: K1.P 13.2,16.54 17.13,12.6 17.13,7.87 18.91,6.66 20.25,5.97 23.54,5.94 24.77,5.97 R11.1 24.91,6.06 24.86,5.97 | 33.18,9 33.17,5.96 33.18,1.92 K15.P | 24.86,6.14 27.8,9.09 33.09,9.09
  Top 2.184: X2.10 49.11,47.72 K11.P@ K11.P 40.77,48.44 K12.P@ 33.42,44.77 33.42,33.94 35.1,32.26 | K13.P K14.P@ | K13.P 35.1,32.26 | K13.P 35.1,32.26 | 35.1,32.26 35.08,32.29 | 35.08,32.29 | 35.08,32.29 33.07,30.68 33.2,14.47 33.18,9
N$47
  Top 1.422: X2.3 50.97,14.73 K16.S
N$48  (via drill 0.7)
  Top 1.422: K2.S 6.93,32.43 5.68,31.18 5.68,18.95 0.84,15.77 0.84,0.79 0.88,0.84 14.25,0.84 16.1,2.73 25.63,2.73 27.49,4.54 27.89,4.76 v30.36,4.76 | X2.1 50.92,4.76 v36.23,4.76
  Bottom 1.422: v36.23,4.76 v30.36,4.76
N$49
  Top 0.305: X4.4 79.21,3.55 81.75,1.7 84.12,1.7 R18.1
  Top 2.184: X4.4 77.94,6.29 76.91,7.32 76.91,12.63 72.97,16.56 K3.P 70.79,19.75 K4.P
N$50
  Top 1.422: K13.S 44.19,19.56 45.12,19.61 45.12,22.83 46.34,24.6 46.37,24.64 52.2,24.64 X2.5
N$51  (via drill 0.7)
  Top 1.422: v36.07,24.71 37.16,27.52 38.91,27.54 54.12,27.54 X2.6
  Bottom 1.422: K14.S 33.78,19.59 33.83,19.63 33.83,22.38 34.44,23.73 35.69,24.5 v36.07,24.71
N$52
  Bottom 1.422: X2.4 51.23,17.07 37.9,17.07 K15.S
N$54
  Bottom 0.305: X4.3 72.91,1.68 74.3,0.29 80.68,0.29 84.9,4.49 84.9,9.87 B1.AC2
N$55
  Top 2.184: X4.2 68.97,5.28 71.89,8.2 72.86,9.12 K3.S
N$56
  Bottom 0.305: R17.2 69.35,9.21 70.93,7.66 74.27,7.66 75.55,8.96 75.55,12.46 IC2.D
N$57  (via drill 0.5)
  Top 0.305: v86.69,0.63 86.81,0.82 86.24,0.25 65.94,0.25 65.39,0.8 65.39,6.75 63.67,8.48 63.67,13.04 C2.+
  Bottom 0.305: R17.1 67.71,16.86 C2.+ | B1.+ 86.2,4.52 87,3.71 87,1.01 v86.69,0.63
N$58
  Bottom 0.305: B1.AC1 86.2,11.22 86.18,11.21 86.18,12.38 R18.2
N$59
  Bottom 0.305: C3.1 77,18.81 76.96,17.93 77.15,17.58 IC2.BP
N$60
  Bottom 0.305: R19.1 77.22,23.69 78.06,24.57 78.71,25.88 C4.+ 79.17,25.91 79.07,26.01 79.07,28.63 D12.C
N$61  (via drill 0.5)
  Top 0.305: K3.2 80.59,13.65 76.47,17.78 76.47,20.94 75.88,21.53 75.87,34.65 75.36,35.1 75.36,36.55 72.18,38.88 72.19,40.68 68.68,44.26 68.31,44.15 v67.66,43.92
  Bottom 0.305: v67.66,43.92 68,44.47 T9.3 67.5,45.7 D13.A
N$62
  Bottom 0.305: T9.1 70.66,45.75 70.66,46.52 70.56,46.62 73.29,46.62 73.39,46.52 R22.2
N$63  (via drill 0.5)
  Top 0.305: v74.12,28.09 75.3,28.9 75.32,34.39 72.79,36.44 69.37,36.43 68.07,37.7 67.96,37.96 67.95,37.99 67.94,38.77 67.56,39.18 65.61,39.18 65.53,39.07 L2.1
  Bottom 0.305: v74.12,28.09 74.16,25.89 C4.- 74.17,24.77 75.62,22.78 75.62,21.45 75.59,20.65 75.16,20.41 C3.2 73.34,15.85 IC2.S 73.37,15.44 78.15,15.4 78.8,14.7 R20.2 79.77,14.1 83.63,16.48 83.64,18.43 83.64,20.93 85.16,20.92 D11.C
N$64  (via drill 0.5)
  Top 0.305: v67.6,40.1 67.23,41.02 65.55,41.03 65.55,41.94 65.56,44.86 68.32,44.84 68.86,44.84 69.58,44.2 74.59,39.14 74.62,39.1 75.15,38.49 77.92,38.49 78.39,38.13 78.39,36.99 78.36,36.98 78.37,34.68 v83.61,29.11
  Bottom 0.305: K4.2 64.36,29.91 64.38,33.87 65.84,35.36 65.86,37.34 65.82,37.96 66.03,38.52 66.39,38.69 67.38,38.73 67.61,38.91 v67.6,40.1 | T10.3 83.39,27.27 D14.A 83.83,29.34 v83.61,29.11
N$65
  Bottom 0.305: R23.2 81.51,45.75 82.72,44.59 82.73,42.51 85.18,42.51 85.18,37.75 87,36.1 87,33.57 87,33.52 87,27.99 86.63,27.64 84.72,27.68 83.28,26.23 T10.1
N$66
  Top 2.184: K4.S 66.71,32.45 65.45,31.2 65.45,18.97 61.01,14.52 61.01,5.44 X4.1
RST  (via drill 0.5)
  Top 0.305: v18.59,32.28 18.59,32.96 17.44,34.17 16.88,34.76 16.88,35.14 16.88,36.91 15.27,38.56 14.55,38.56 9.5,44.64 7.23,44.64 v6.99,43.9
  Bottom 0.305: 17.12,33.57 ATMEGA328.29 17.12,33.57 | 17.12,33.57 17.42,33.27 17.42,32.51 R1.2 | U$2.VPP 9.2,49.19 7.91,49.19 7.24,48.52 RESET.1 4.6,48.54 4.6,43.9 v6.99,43.9 | 17.12,33.57 18.32,32.37 18.62,32.37 v18.59,32.28
RST1  (via drill 0.5)
  Top 0.305: U$6.VPP 86.56,34.58 85.5,34.57 81.89,34.57 v81.52,34.38
  Bottom 0.305: ATMEGA1.29 76.89,33.6 77.2,33.29 | 77.2,33.29 77.2,32.53 R16.2 | v81.52,34.38 81.35,34.4 80.59,33.57 77.55,33.57 77.2,33.29 | 83.95,43.3 RESET1.1 85.72,43.96 85.73,43.3 85.73,38.4 U$6.VPP
VCC  (via drill 0.5, 0.6)
  Top 0.305: v10.6,25.03 12.37,26.36 12.38,28.65 12.38,30.6 v13.97,32.45 13.43,32.95 10.71,35.66 9.41,35.67 7.53,37.53 7.53,38.28 7.07,38.59 6.31,38.6 5.96,38.39 5.25,37.59 4.7,37.36 4.02,37.49 3.59,37.94 3.62,40.56 3.7,40.67 4.03,41.31 v3.73,42.34 | U$5.VDD 26.44,25.75 v22.52,30.25 22.55,31.44 v20.4,31.44 | v16.7,38.34 17.69,37.1 17.7,35.76 v19.54,33.14
  Bottom 0.305: IC3.4 5.32,25.03 | 5.32,25.03 IC3.2 9.51,25.03 v10.6,25.03 | ATMEGA328.6 14.26,40.08 | 14.26,40.08 14.45,40.12 15.12,40.82 15.97,40.82 16.49,41.46 18.3,41.46 18.32,41.44 18.34,41.44 18.85,40.93 21.79,40.9 ATMEGA328.18 | 14.26,40.08 14.45,39.89 14.45,39.03 13.89,38.48 ATMEGA328.4 v16.7,38.34 | v13.97,32.45 15.75,32.48 R1.1 15.82,32.47 16.19,31.44 18.64,31.44 19.53,31.44 | v22.52,30.25 22.53,31.39 C10.2 | 19.53,31.44 v20.4,31.44 | JP1.1 3.98,45.54 3.97,42.67 v3.73,42.34 | v19.54,33.14 19.54,31.45 19.53,31.44 | C11.+ 1.93,15.71 5.38,19.21 5.38,24.97 5.32,25.03
VCC1  (via drill 0.5)
  Top 0.305: v71.1,25.48 72.14,26.38 72.16,28.67 72.16,30.09 v73.84,32.51 72.16,35.19 arc61 70.59,35.89 69.21,35.82 67.46,37.62 67.46,38.38 67.12,38.66 66.34,38.69 66,38.58 65.83,38.25 65.65,37.65 64.84,37.47 64.03,37.47 63.73,37.66 63.37,38.11 63.37,40.58 63.48,40.69 v63.46,41.63 | v75.96,37.64 75.96,35.5 76.43,34.96 76.45,32.58 v79.08,32.59 | v79.04,30.65 79.32,30.15 82.03,27.44 86.22,27.42 86.22,27.36 U$4.VDD v82.06,16.74
  Bottom 0.305: IC4.4 IC4.2 70.67,25.05 v71.1,25.48 | ATMEGA1.6 74.09,39.98 | 74.09,39.98 74.29,40.02 75.05,40.02 76.39,40.02 76.92,40.79 77.56,40.79 77.9,40.78 78.11,40.8 78.24,40.8 81.57,40.8 ATMEGA1.18 | 74.09,39.98 74.22,39.91 74.22,39.05 73.67,38.5 ATMEGA1.4 75.1,38.5 75.1,38.27 v75.96,37.64 | v73.84,32.51 75.53,32.5 R16.1 75.6,32.49 75.65,31.36 79.08,31.32 | 79.08,31.32 v79.04,30.65 | 79.08,31.32 v79.08,32.59 79.06,32.45 80.27,32.45 80.3,32.49 C13.2 | JP2.1 63.11,43.78 v63.46,41.63 | C12.+ v82.06,16.74
XXX
  Bottom 0.305: IC1.FB 18.18,16.25 19.44,16.28 19.69,16.28 R13.1 20,16 R12.2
